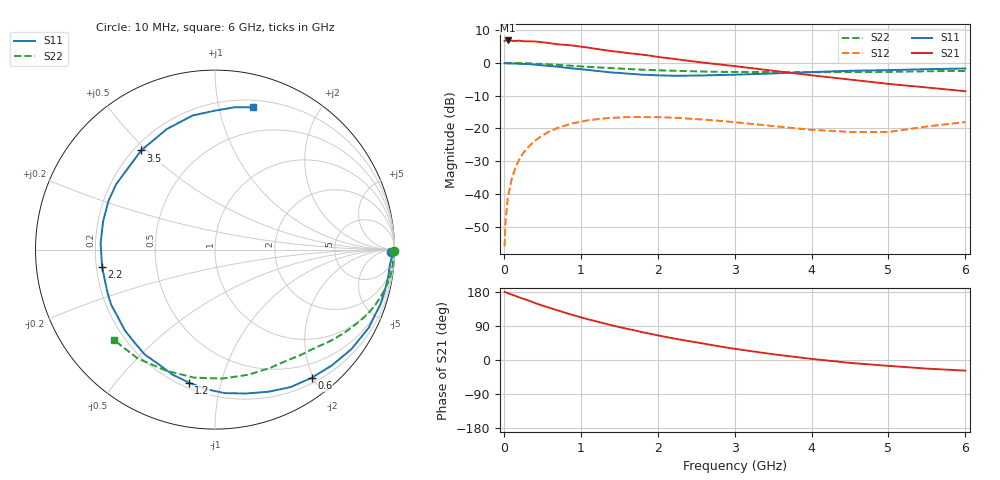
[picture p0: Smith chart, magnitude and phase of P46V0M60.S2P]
! SIEMENS Small Signal Semiconductors
! BFP182
! Si NPN RF Bipolar Junction Transistor in SOT143
! VCE = 6 V  IC = 0.6 mA
! Common Emitter S-Parameters:  March  1996
# GHz  S  MA  R  50
!  f  S11  S21  S12  S22
! GHz  MAG  ANG  MAG  ANG  MAG  ANG  MAG  ANG
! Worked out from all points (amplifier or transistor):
!   36 points, 10 MHz to 6 GHz, reference 50 ohm
!   highest |S21| = 6.8 dB at 50 MHz (marker M1)
!   |S21| within 3 dB of that: start of sweep to 1.326 GHz
!   unconditionally stable (mu >= 1): 2.898 GHz to end of sweep
!   at 250 MHz: K = 0.09, MSG = 17.1 dB, |S12| = -27.6 dB
!   at 1.4 GHz: K = 0.50, MSG = 10.2 dB, |S12| = -16.8 dB
!   at 6 GHz: K = 1.16, MAG = 2.3 dB, |S12| = -18.1 dB
!   S11 on the Smith chart (normalised r, x): 10 MHz: 63, -53; 600 MHz: 0.28, -1.97; 1.2 GHz: 0.23, -0.79; 2.2 GHz: 0.22, -0.07; 3.5 GHz: 0.23, +0.48; 6 GHz: 0.26, +1.26
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0.01  0.9816 -0.9  2.171 179.6  0.0016 94.0  0.9989 -0.3
0.02  0.989 -1.9  2.182 179.2  0.0035 83.3  0.9999 -0.7
0.05  0.9788 -4.6  2.196 176.4  0.0085 91.6  0.9983 -1.6
0.1  0.977 -8.9  2.173 172.8  0.0165 83.0  0.9941 -3.2
0.15  0.9735 -13.8  2.157 169.2  0.0253 81.4  0.9943 -4.9
0.2  0.9704 -18.4  2.179 165.3  0.0334 78.2  0.9919 -6.5
0.25  0.9627 -22.5  2.139 161.8  0.0415 75.5  0.9887 -8.3
0.4  0.9409 -36.1  2.12 150.8  0.0644 67.0  0.974 -12.8
0.6  0.8947 -53.0  1.993 137.4  0.0911 55.7  0.9466 -18.6
0.9  0.8202 -77.8  1.834 118.5  0.1199 41.3  0.8997 -26.2
1.1  0.7788 -93.9  1.709 107.1  0.1331 32.8  0.8693 -30.7
1.2  0.7551 -101.2  1.633 102.1  0.1377 28.7  0.8564 -32.9
1.5  0.7035 -123.8  1.469 86.9  0.1465 18.5  0.819 -38.4
1.8  0.6585 -145.4  1.334 73.4  0.1495 10.2  0.7865 -43.5
2.2  0.6367 -171.2  1.155 57.2  0.146 0.7  0.7591 -50.3
2.8  0.6524 155.7  0.946 36.0  0.1307 -9.0  0.7298 -60.9
3.5  0.6889 126.7  0.758 15.2  0.1087 -13.5  0.7215 -75.2
4  0.7232 111.8  0.646 2.9  0.0952 -9.9  0.7196 -86.8
4.5  0.7574 99.5  0.556 -7.6  0.0885 -2.9  0.7228 -99.3
5  0.7742 90.0  0.478 -15.5  0.0882 10.0  0.7278 -112.1
5.5  0.8007 82.1  0.421 -22.7  0.1071 15.0  0.7439 -125.4
6  0.82 75.2  0.369 -28.1  0.1248 16.0  0.7556 -138.2
